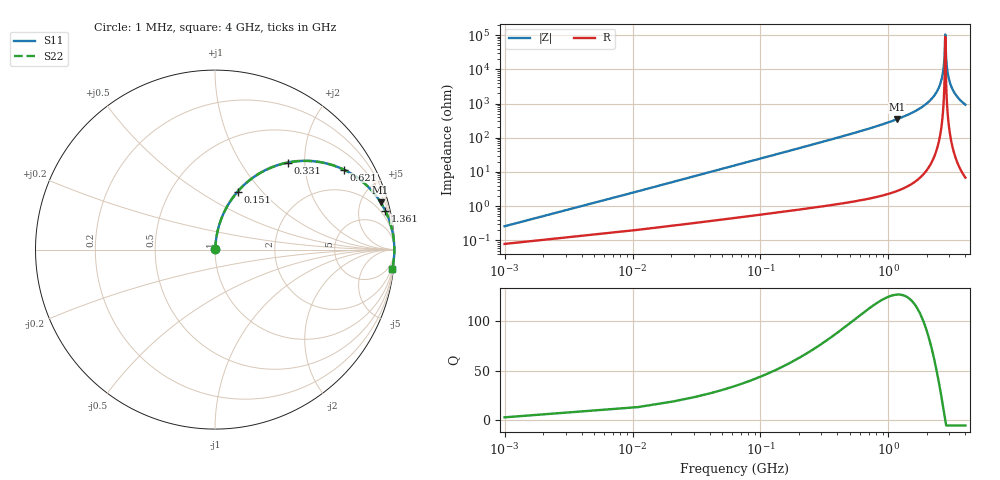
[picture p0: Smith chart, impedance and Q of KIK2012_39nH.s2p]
!version-2
!date-01.2022
!Series
# MHz S RI R 50
!Freq ReS11 ImS11 ReS21 ImS21 ReS12 ImS12 ReS22 ImS22
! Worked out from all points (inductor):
!   401 points, 1 MHz to 4 GHz, reference 50 ohm
!   read as one part in series: L = 39 nH near 21 MHz
!   highest Q = 126 at 1.171 GHz (marker M1), where L = 47.4 nH
!   self-resonance near 2.781 GHz
!   S11 on the Smith chart (normalised r, x): 1 MHz: 1.00, +0.00; 151 MHz: 1.01, +0.74; 331 MHz: 1.02, +1.65; 621 MHz: 1.03, +3.20; 1.361 GHz: 1.07, +8.76; 4 GHz: 1, -18
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1  0.000786 0.00245  0.9992 -0.00245  0.9992 -0.00245  0.000786 0.00245
31  0.00889 0.0751  0.9911 -0.0751  0.9911 -0.0751  0.00889 0.0751
41  0.0135 0.0988  0.9865 -0.0988  0.9865 -0.0988  0.0135 0.0988
81  0.0424 0.1893  0.9576 -0.1893  0.9576 -0.1893  0.0424 0.1893
151  0.1256 0.3223  0.8744 -0.3223  0.8744 -0.3223  0.1256 0.3223
331  0.4048 0.4847  0.5952 -0.4847  0.5952 -0.4847  0.4048 0.4847
621  0.7176 0.4455  0.2824 -0.4455  0.2824 -0.4455  0.7176 0.4455
671  0.7509 0.4279  0.2491 -0.4279  0.2491 -0.4279  0.7509 0.4279
1171  0.9222 0.264  0.0778 -0.264  0.0778 -0.264  0.9222 0.264
1341  0.9466 0.2209  0.0534 -0.2209  0.0534 -0.2209  0.9466 0.2209
1361  0.9489 0.2162  0.0511 -0.2162  0.0511 -0.2162  0.9489 0.2162
2001  0.9893 0.0975  0.0107 -0.0975  0.0107 -0.0975  0.9893 0.0975
2441  0.9976 0.0387  0.0024 -0.0387  0.0024 -0.0387  0.9976 0.0387
2671  0.999 0.0123  0.000992 -0.0123  0.000992 -0.0123  0.999 0.0123
2721  0.9991 0.00687  0.000878 -0.00687  0.000878 -0.00687  0.9991 0.00687
2771  0.9992 0.00154  0.000824 -0.00154  0.000824 -0.00154  0.9992 0.00154
2791  0.9992 -0.000564  0.000818 0.000564  0.000818 0.000564  0.9992 -0.000564
2851  0.9991 -0.00679  0.000854 0.00679  0.000854 0.00679  0.9991 -0.00679
2941  0.999 -0.0159  0.00105 0.0159  0.00105 0.0159  0.999 -0.0159
3101  0.9982 -0.0314  0.00177 0.0314  0.00177 0.0314  0.9982 -0.0314
3341  0.9964 -0.0533  0.00362 0.0533  0.00362 0.0533  0.9964 -0.0533
4000  0.9876 -0.1069  0.0124 0.1069  0.0124 0.1069  0.9876 -0.1069
